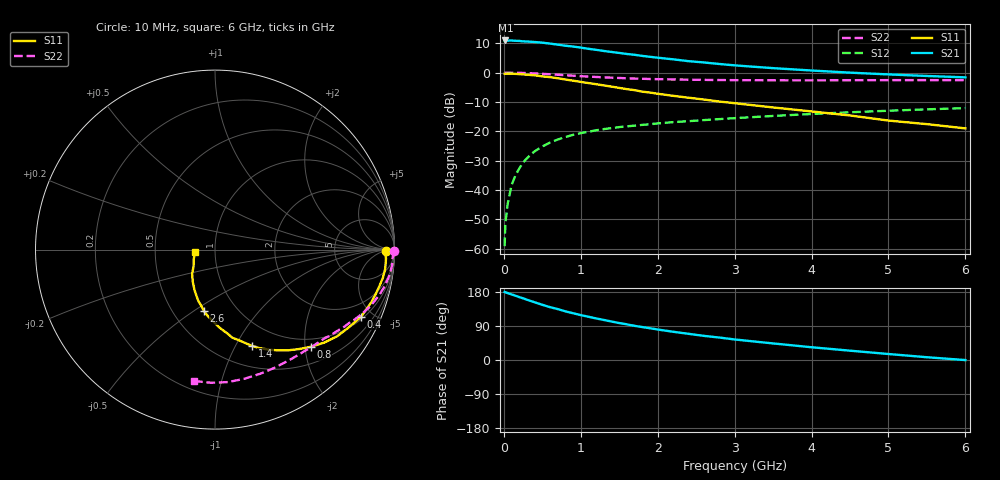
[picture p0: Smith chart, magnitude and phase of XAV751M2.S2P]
! SIEMENS Discrete & RF Semiconductors
! BFY180
! Si NPN RF Bipolar Junction Transistor in MICRO-X
! VCE = 0.75 V  IC = 1.2 mA
! Common Emitter S-Parameters:  May  1997
# GHz  S  MA  R  50
!  f  S11  S21  S12  S22
! GHz  MAG  ANG  MAG  ANG  MAG  ANG  MAG  ANG
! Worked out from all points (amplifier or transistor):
!   36 points, 10 MHz to 6 GHz, reference 50 ohm
!   highest |S21| = 10.9 dB at 20 MHz (marker M1)
!   |S21| within 3 dB of that: start of sweep to 1.145 GHz
!   unconditionally stable (mu >= 1): 2.341 GHz to end of sweep
!   at 250 MHz: K = 0.13, MSG = 20.7 dB, |S12| = -30.7 dB
!   at 1.4 GHz: K = 0.72, MSG = 13.0 dB, |S12| = -18.9 dB
!   at 6 GHz: K = 1.18, MAG = 2.7 dB, |S12| = -12.1 dB
!   S11 on the Smith chart (normalised r, x): 10 MHz: 38, -7; 400 MHz: 1.13, -4.30; 800 MHz: 0.83, -2.12; 1.4 GHz: 0.73, -1.17; 2.6 GHz: 0.71, -0.55; 6 GHz: 0.80, -0.02
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0.01  0.9506 -0.5  3.472 179.6  0.0011 80.8  0.9953 -0.3
0.02  0.9496 -1.3  3.517 178.6  0.0027 91.9  0.9949 -0.6
0.05  0.954 -3.0  3.492 176.7  0.0058 88.2  0.9932 -1.6
0.1  0.9543 -6.4  3.51 173.2  0.012 86.8  0.99 -3.3
0.15  0.9483 -9.6  3.472 169.7  0.0176 83.8  0.9912 -4.9
0.25  0.9284 -15.6  3.395 162.8  0.0292 79.8  0.9835 -8.1
0.4  0.8963 -24.6  3.307 152.4  0.0454 73.3  0.9652 -12.6
0.5  0.8602 -30.5  3.228 145.7  0.0549 69.6  0.9497 -15.4
0.6  0.8343 -35.4  3.109 139.5  0.064 66.2  0.9332 -18.0
0.8  0.7603 -45.4  2.861 128.4  0.0796 59.8  0.8994 -22.8
0.9  0.7261 -49.7  2.771 123.4  0.0867 56.9  0.8831 -24.9
1.1  0.6605 -58.2  2.534 114.1  0.0979 52.6  0.8518 -28.7
1.4  0.5753 -68.9  2.238 101.5  0.1129 46.9  0.8159 -34.0
1.7  0.5006 -78.8  2.003 90.1  0.1243 43.1  0.7875 -38.6
2  0.4346 -86.8  1.788 80.5  0.1359 39.8  0.7709 -42.9
2.2  0.4011 -91.4  1.678 74.5  0.1428 37.5  0.7624 -45.9
2.6  0.3467 -100.3  1.484 63.7  0.1546 34.2  0.7488 -51.2
3  0.3002 -108.1  1.324 54.2  0.1669 31.0  0.7414 -56.6
3.5  0.2541 -116.6  1.187 43.7  0.182 27.5  0.7372 -63.4
4.5  0.1854 -133.4  0.995 24.6  0.2102 19.4  0.7379 -77.1
5.5  0.1319 -154.7  0.873 7.3  0.2358 10.9  0.7423 -91.7
6  0.1117 -172.9  0.827 -0.2  0.2475 6.4  0.741 -98.9
